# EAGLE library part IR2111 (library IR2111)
MOSFET/IGBT driver IR2111 DIP8 200mA Source: Datasheet
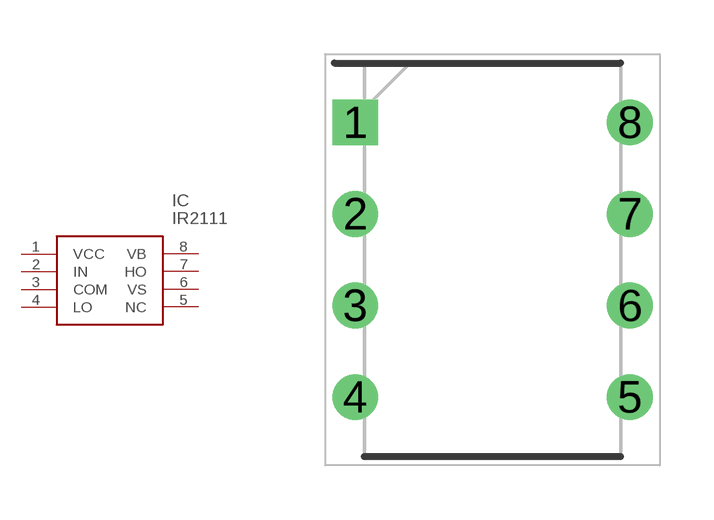
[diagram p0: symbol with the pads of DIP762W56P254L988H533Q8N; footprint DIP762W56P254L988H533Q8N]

Designator prefix IC

## IR2111 (Description: MOSFET/IGBT driver IR2111 DIP8 200mA; Height: 5.33mm; Manufacturer_Name: Infineon; Manufacturer_Part_Number: IR2111)  [DIP762W56P254L988H533Q8N]
1  VCC  pwr
2  IN  in
3  COM  pwr
4  LO  out
5  NC  nc
6  VS  pwr
7  HO  out
8  VB  pwr

## Footprint DIP762W56P254L988H533Q8N (pad centres in mm)
DIP-8
drill 0.758 pad 1.158 square: 1 -3.81,3.81
drill 0.758 pad 1.158: 2 -3.81,1.27; 3 -3.81,-1.27; 4 -3.81,-3.81; 5 3.81,-3.81; 6 3.81,-1.27; 7 3.81,1.27; 8 3.81,3.81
